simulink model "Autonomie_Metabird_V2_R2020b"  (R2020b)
settings: Solver=VariableStepAuto  StartTime=0.0  StopTime=450  RelTol=1e-3
model workspace (MAT data in the model file):
  Q = 1
undefined symbols (not defined in the file): set
libraries: fl_lib x7, nesl_utility x5, ee_lib x2

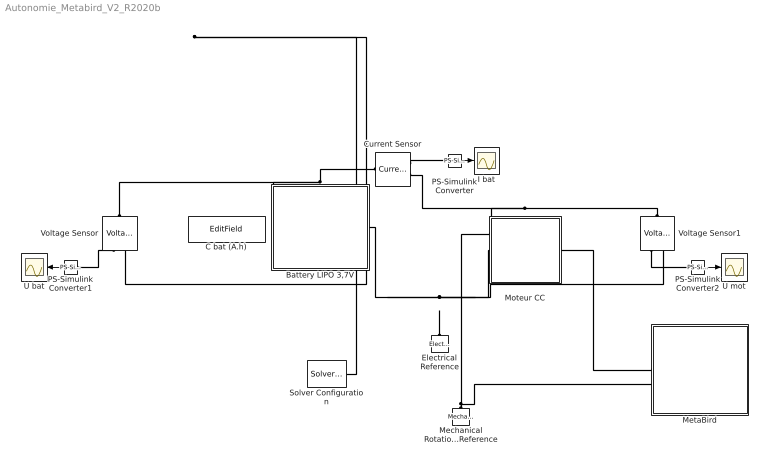
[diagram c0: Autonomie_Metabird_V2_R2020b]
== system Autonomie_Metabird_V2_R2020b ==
  Battery LIPO 3,7V : Subsystem
  C bat (A.h) : EditField  Description=EEE  LabelPosition=Hide  ShowInitialText=on  Alignment=Center
  Current Sensor : fl_lib/Electrical/Electrical Sensors/Current Sensor
  Electrical Reference : fl_lib/Electrical/Electrical Elements/Electrical Reference
  I bat : Scope
  Mechanical Rotational Reference : fl_lib/Mechanical/Rotational Elements/Mechanical Rotational Reference
  MetaBird : Subsystem
  Moteur CC : Subsystem
  PS-Simulink Converter : nesl_utility/PS-Simulink Converter  PhysicalDomain=network_engine_domain  SubClassName=ps_output  LeftPortType=input  RightPortType=output  PseudoPeriodic=off  Frequencies=[]  Unit=mA  AffineConversion=off
  PS-Simulink Converter1 : nesl_utility/PS-Simulink Converter  PhysicalDomain=network_engine_domain  SubClassName=ps_output  LeftPortType=input  RightPortType=output  PseudoPeriodic=off  Frequencies=[]  Unit=V  AffineConversion=off
  PS-Simulink Converter2 : nesl_utility/PS-Simulink Converter  PhysicalDomain=network_engine_domain  SubClassName=ps_output  LeftPortType=input  RightPortType=output  PseudoPeriodic=off  Frequencies=[]  Unit=V  AffineConversion=off
  Solver Configuration : nesl_utility/Solver Configuration  PhysicalDomain=network_engine_domain  SubClassName=solver  LeftPortType=input  RightPortType=generic  Tones=[]  Harmonics=[]  SimulateNoise=off  Profile=off  UseLocalSampling=off  EnableSwitchedLinearOptims=on  FrequencyDomain=off  UseCCode=off  RelTol=0.001  AbsTol=0.001  MinStep=1e-09  ToWorkspace=off  RevertToSquareIcSolve=off  NumHomotopyIterations=100  PhasorMode=off  PhasorModeNumHarmonics=1  DoDC=off  ResidualTolerance=1e-09  UseLocalSolver=off  LocalSolverChoice=NE_BACKWARD_EULER_ADVANCER  LocalSolverSampleTime=0.001  DoFixedCost=off  MaxNonlinIter=3  MaxModeIter=2  ComputeImpulses=off  ImpulseIterations=2  LinearAlgebra=auto  EquationFormulation=NE_TIME_EF  DelaysMemoryBudget=1024  AutomaticFiltering=on  FilteringTimeConstant=0.001  PartitionStorageMethod=AS_NEEDED  PartitionMemoryBudget=1024  PartitionMethod=ROBUST
  U bat : Scope
  U mot : Scope
  Voltage Sensor : fl_lib/Electrical/Electrical Sensors/Voltage Sensor
  Voltage Sensor1 : fl_lib/Electrical/Electrical Sensors/Voltage Sensor
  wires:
  PS-Simulink Converter/1 -> I bat/1
  PS-Simulink Converter1/1 -> U bat/1
  PS-Simulink Converter2/1 -> U mot/1
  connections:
  Voltage Sensor/LConn1 -- Current Sensor/LConn1 -- Battery LIPO 3,7V/LConn1
  Voltage Sensor1/LConn1 -- Moteur CC/LConn3 -- Current Sensor/RConn2
  Electrical Reference/LConn1 -- Voltage Sensor1/RConn2 -- Moteur CC/LConn2 -- Voltage Sensor/RConn2 -- Solver Configuration/RConn1 -- Battery LIPO 3,7V/RConn1
  Current Sensor/RConn1 -- PS-Simulink Converter/LConn1
  PS-Simulink Converter1/LConn1 -- Voltage Sensor/RConn1
  Voltage Sensor1/RConn1 -- PS-Simulink Converter2/LConn1
  Moteur CC/RConn1 -- MetaBird/LConn1
  Mechanical Rotational Reference/LConn1 -- MetaBird/LConn2 -- Moteur CC/LConn1

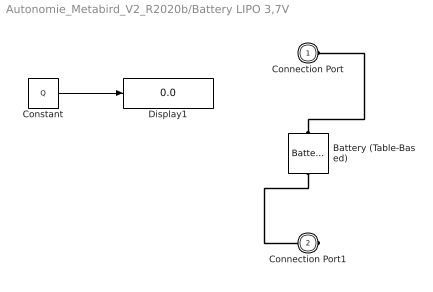
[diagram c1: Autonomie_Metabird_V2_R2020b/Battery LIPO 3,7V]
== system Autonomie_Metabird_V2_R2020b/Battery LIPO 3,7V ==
  Battery (Table-Based) : ee_lib/Sources/Battery (Table-Based)  Tag={'toolbox/physmod/elec/library/m/ee_lib_parts';'Sources/Battery__Table_Based_/Korea_Powercell/PD3032.xml'}  SOC_vec="[0 0.01 0.02 0.03 0.04 0.05 0.06 0.07 0.08 0.09 0.1 0.11 0.12 0.13 0.14 0.15 0.16 0.17 0.18 0.19 0.2 0.21 0.22 0.23 0.24 0.25 0.26 0.27 0.28 0.29 0.3 0.31 0.32 0.33 0.34 0.35 0.36 0.37 0.38 0.39 0.4 0.41 0.42 0.43 0.44 0.45 0.46 0.47 0.48 0.49 0.5 0.51 0.52 0.53 0.54 0.55 0.56 0.57 0.58 0.59 0.6 0.61 0.62 0.63 0.64 0.65 0.66 0.67 0.68 0.69 0.7 0.71 0.72 0.73 0.74 0.75 0.76 0.77 0.78 0.79 0.8 0.81 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"  T_dependence=ee.enum.temperature_dependence.no  prm_dir=ee.enum.battery.prm_dir.noCurrentDirectionality  T_vec=[-20 -10 25] degC  V0_mat=[2.95724 3.3564 3.49366 3.58258 3.63766 3.68332 3.70873 3.73055 3.74166 3.74045 3.73776 3.73631 3.73521 3.73661 3.73787 3.73862 3.74076 3.74303 3.74502 3.7472 3.74981 3.75229 3.7538 3.75584 3.75779 3.75969 3.76148 3.76318 3.76489 3.76695 3.76868 3.77025 3.77183 3.77343 3.77506 3.77658 3.77841 3.78029 3.78217 3.78415 3.78659 3.78921 3.79241 3.7956 3.79881 3.80207 3.80534 3.80863 3.81212 3.81572 3.8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  V0_vec=[2.95724 3.3564 3.49366 3.58258 3.63766 3.68332 3.70873 3.73055 3.74166 3.74045 3.73776 3.73631 3.73521 3.73661 3.73787 3.73862 3.74076 3.74303 3.74502 3.7472 3.74981 3.75229 3.7538 3.75584 3.75779 3.75969 3.76148 3.76318 3.76489 3.76695 3.76868 3.77025 3.77183 3.77343 3.77506 3.77658 3.77841 3.78029 3.78217 3.78415 3.78659 3.78921 3.79241 3.7956 3.79881 3.80207 3.80534 3.80863 3.81212 3.81572 3.8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  R0_mat=[0.86823 1.97565 2.19839 2.30336 2.32493 2.32311 2.27325 2.21593 2.13322 2.00795 1.88032 1.79212 1.70777 1.65332 1.59953 1.54628 1.51052 1.47625 1.44119 1.41044 1.38852 1.36656 1.34119 1.32173 1.30512 1.28839 1.27179 1.25526 1.23874 1.2262 1.21367 1.20059 1.1875 1.17438 1.1611 1.14754 1.13738 1.12789 1.11839 1.10879 1.10081 1.09337 1.08812 1.08292 1.0777 1.07242 1.06713 1.0619 1.0576 1.05404 1.051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  R0_vec=[0.86823 1.97565 2.19839 2.30336 2.32493 2.32311 2.27325 2.21593 2.13322 2.00795 1.88032 1.79212 1.70777 1.65332 1.59953 1.54628 1.51052 1.47625 1.44119 1.41044 1.38852 1.36656 1.34119 1.32173 1.30512 1.28839 1.27179 1.25526 1.23874 1.2262 1.21367 1.20059 1.1875 1.17438 1.1611 1.14754 1.13738 1.12789 1.11839 1.10879 1.10081 1.09337 1.08812 1.08292 1.0777 1.07242 1.06713 1.0619 1.0576 1.05404 1.051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  R0_dis_mat=[0.03 0.015 0.002;0.04 0.017 0.008;0.039 0.012 0.006;0.027 0.013 0.021] % Parameter not set Ohm  R0_dis_vec=[0.015 0.017 0.012 0.013] % Parameter not set Ohm  R0_ch_mat=[0.03 0.015 0.002;0.04 0.017 0.008;0.039 0.012 0.006;0.027 0.013 0.021] % Parameter not set Ohm  R0_ch_vec=[0.015 0.017 0.012 0.013] % Parameter not set Ohm  AH_vec=[0.058 0.058 0.058] hr*A  AH=Q+Q*0.15 hr*A  prm_leak=ee.enum.battery.prm_leak.disabled  Rleak_vec=[8000 7000 6000] % Parameter not set Ohm  Rleak=7000 % Parameter not set Ohm  extrapolation_option=ee.enum.extrapolation.nearest  prm_dyn=ee.enum.battery.prm_dyn.off  R1_mat=[0.089 0.076 0.01;0.042 0.022 0.099;0.019 0.007 0.002;0.051 0.043 0.029] % Parameter not set Ohm  R1_vec=[0.076 0.022 0.007 0.043] % Parameter not set Ohm  tau1_mat=[44 148 235;93 110 1000;19 27 133;0.5 22 3] % Parameter not set s  tau1_vec=[148 110 27 22] % Parameter not set s  R2_mat=[0.014 0.382 0.407;0.028 0.006 0.007;0.014 0.007 0.006;0.333 0.956 0.912] % Parameter not set Ohm  R2_vec=[0.382 0.006 0.007 0.956] % Parameter not set Ohm  tau2_mat=[1 44 5644;11 24 506;2 14 330;3310 13419 30216] % Parameter not set s  tau2_vec=[44 24 14 13419] % Parameter not set s  R3_mat=[0.014 0.382 0.407;0.028 0.006 0.007;0.014 0.007 0.006;0.333 0.956 0.912] % Parameter not set Ohm  R3_vec=[0.382 0.006 0.007 0.956] % Parameter not set Ohm  tau3_mat=[1 44 5644;11 24 506;2 14 330;3310 13419 30216] % Parameter not set s  tau3_vec=[44 24 14 13419] % Parameter not set s  R4_mat=[0.014 0.382 0.407;0.028 0.006 0.007;0.014 0.007 0.006;0.333 0.956 0.912] % Parameter not set Ohm  R4_vec=[0.382 0.006 0.007 0.956] % Parameter not set Ohm  tau4_mat=[1 44 5644;11 24 506;2 14 330;3310 13419 30216] % Parameter not set s  tau4_vec=[44 24 14 13419] % Parameter not set s  R5_mat=[0.014 0.382 0.407;0.028 0.006 0.007;0.014 0.007 0.006;0.333 0.956 0.912] % Parameter not set Ohm  R5_vec=[0.382 0.006 0.007 0.956] % Parameter not set Ohm  tau5_mat=[1 44 5644;11 24 506;2 14 330;3310 13419 30216] % Parameter not set s  tau5_vec=[44 24 14 13419] % Parameter not set s  prm_fade=ee.enum.battery.prm_fade.tableN  N0=100 % Parameter not set  dV0=0 % Parameter not set  dR0=0 % Parameter not set  dAH=0 % Parameter not set  dRleak=0 % Parameter not set  dR1=0 % Parameter not set  dR2=0 % Parameter not set  dR3=0 % Parameter not set  dR4=0 % Parameter not set  dR5=0 % Parameter not set  N0vec=[1 7 13 19 25 31 37 43 49 55 61 67 73 79 85 91 97 103 109 115 121 127 133 139 145 151 157 163 169 175 181 187 193 199 205 211 217 223 229 235 241 247 253 259 265 271 277 283 289 295 301 307 313 319 325 331 337 343 349 355 361 367 373 379 385 391 397 403 409 415 421 427 433 439 445 451 457 463 469 475 481 487 493 499]  Tfadevec=[298.15 323.15] % Parameter not set K  dV0vec=[0 -0.0628438826149197 -0.125687765229839 -0.18853164784478 -0.251375530459721 -0.314219413074662 -0.377063295689582 -0.451508979909996 -0.562003276816908 -0.667452593509906 -0.772901910202884 -0.878351226895861 -0.96290491111089 -1.04466751936566 -1.12332313736417 -1.20197875536267 -1.26256181580412 -1.3222060579416 -1.38185030007906 -1.44149454221653 -1.50255421857852 -1.56371974345091 -1.624885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  dR0vec=[0;0;0;0;0;0;0;0;0;0;0;0;0;0;0;0;0;0;0;0;0;0;0;0;0;0;0;0;0;0;0;0;0;0;0;0;0;0;0;0;0;0;0;0;0;0;0;0;0;0;0;0;0;0;0;0;0;0;0;0;0;0;0;0;0;0;0;0;0;0;0;0;0;0;0;0;0;0;0;0;0;0;0;0] % Parameter not set  dAHvec=[0 -0.130046736538462 -0.260093473076939 -0.39014020961543 -0.520186946153922 -0.650233682692399 -0.780280419230876 -0.934335482021324 -1.19380012181077 -1.45326476160023 -1.71272940138966 -1.9721940411791 -2.23165868096855 -2.49022842430935 -2.73897248216537 -2.9877165400214 -3.23646059787742 -3.48520465573346 -3.73394871358948 -3.9826927714455 -4.23143682930151 -4.48018088715753 -4.7289249450135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  dRleakvec=[0 0 0] % Parameter not set  dR1vec=[0 0 0] % Parameter not set  dR2vec=[0 0 0] % Parameter not set  dR3vec=[0 0 0] % Parameter not set  dR4vec=[0 0 0] % Parameter not set  dR5vec=[0 0 0] % Parameter not set  dV0mat=[0 0;0 0;0 0] % Parameter not set  dR0mat=[0 0;0 0;0 0] % Parameter not set  dAHmat=[0 0;0 0;0 0] % Parameter not set  dRleakmat=[0 0;0 0;0 0] % Parameter not set  dR1mat=[0 0;0 0;0 0] % Parameter not set  dR2mat=[0 0;0 0;0 0] % Parameter not set  dR3mat=[0 0;0 0;0 0] % Parameter not set  dR4mat=[0 0;0 0;0 0] % Parameter not set  dR5mat=[0 0;0 0;0 0] % Parameter not set  temperature=298.15 K  i_specify=off  i_priority=None  i=0 A  i_nominal_specify=off  i_nominal_unit=A  i_nominal_value=1  v_specify=off  v_priority=None  v=0 V  v_nominal_specify=off  v_nominal_unit=V  v_nominal_value=1  stateOfCharge_specify=on  stateOfCharge_priority=High  stateOfCharge=1  stateOfCharge_nominal_specify=off  stateOfCharge_nominal_unit=1  stateOfCharge_nominal_value=1  num_cycles_specify=off  num_cycles_priority=High  num_cycles=0  num_cycles_nominal_specify=off  num_cycles_nominal_unit=1  num_cycles_nominal_value=1  thermal_mass=30000 J/K  temperature_specify=off  temperature_priority=High  temperature_nominal_specify=off  temperature_nominal_unit=K  temperature_nominal_value=1
  Constant : Constant  Value=Q
  Display1 : Display
  Connection Port : PMIOPort  Side=Left
  Connection Port1 : PMIOPort  Port=2  Side=Right
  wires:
  Constant/1 -> Display1/1
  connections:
  Battery (Table-Based)/RConn1 -- Connection Port1/RConn1
  Battery (Table-Based)/LConn1 -- Connection Port/RConn1

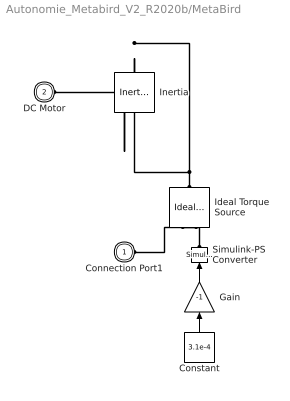
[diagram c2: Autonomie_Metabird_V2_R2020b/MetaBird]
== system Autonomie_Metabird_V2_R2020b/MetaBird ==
  Constant : Constant  Value=3.1e-4
  Gain : Gain  Gain=-1
  Ideal Torque Source : fl_lib/Mechanical/Mechanical Sources/Ideal Torque Source
  Inertia : fl_lib/Mechanical/Rotational Elements/Inertia  inertia=1.91e-8 kg*m^2  num_ports=foundation.enum.numPorts2.one  w_specify=off  w_priority=High  w=0 rad/s  w_nominal_specify=off  w_nominal_unit=rad/s  w_nominal_value=1  t_specify=off  t_priority=None  t=0 N*m  t_nominal_specify=off  t_nominal_unit=N*m  t_nominal_value=1
  Simulink-PS Converter : nesl_utility/Simulink-PS Converter  PhysicalDomain=network_engine_domain  SubClassName=ps_input  LeftPortType=input  RightPortType=output  PseudoPeriodic=off  Frequencies=[]  NoiseDistribution=none  NoiseParameters=[]  Unit=N*m  AffineConversion=off  FilteringAndDerivatives=provide  SimscapeFilterOrder=1  InputFilterTimeConstant=0.001  UdotUserProvided=0
  Connection Port1 : PMIOPort  Side=Left
  DC Motor : PMIOPort  Port=2  Side=Left
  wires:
  Constant/1 -> Gain/1
  Gain/1 -> Simulink-PS Converter/1
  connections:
  Ideal Torque Source/LConn1 -- DC Motor/RConn1 -- Inertia/LConn1
  Simulink-PS Converter/RConn1 -- Ideal Torque Source/RConn1
  Connection Port1/RConn1 -- Ideal Torque Source/RConn2

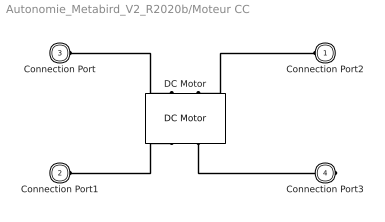
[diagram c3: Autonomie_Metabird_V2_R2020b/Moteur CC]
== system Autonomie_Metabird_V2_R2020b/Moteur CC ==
  DC Motor : ee_lib/Electromechanical/Brushed Motors/DC Motor  field_option=ee.enum.field_option.pm  Rf=100 Ohm  Lf=1 H  Laf=0.15 H  If0=0 A  parameterization=ee.enum.dcparam_option.load_speed  Ra=3.9 Ohm  La=12e-6 H  emf_or_torque=ee.enum.emf_or_torque.kv  Kv=0.072e-3 V/rpm  Ki=6.876e-4 N*m/A  T_stall=0.24e-3 N*m  w_max=53000 rpm  w_rated=37000 rpm  P_rated=1.6 W  V_rated=3.7 V  J=0 g*cm^2  lam_param=ee.enum.lam_param.current  lam=0 N*m/(rad/s)  i_noload=68.1 mA  V_i_noload=3.7 V  speed0=0 rpm  enable_fault_armature=ee.enum.faults.faultEnable.no  rev_faulted=1 / 3  G_faulted_armature=1e-5 S  fault_trigger_armature=ee.enum.faults.faultTrigger.temporal  t_fault_armature=1 s  max_permissible_current_armature=inf A  t_fail_on_current_armature=1 s  enable_fault_field=ee.enum.faults.faultEnable.no  G_faulted_field=1e-5 S  fault_trigger_field=ee.enum.faults.faultTrigger.temporal  t_fault_field=1 s  max_permissible_current_field=inf A  t_fail_on_current_field=1 s  fault_action=ee.enum.faults.faultAction.none  alpha=3.93e-3 1/K  Tmeas=25 degC  thermal_mass=100 J/K  initial_temperature=25 degC
  Connection Port2 : PMIOPort  Side=Left
  Connection Port1 : PMIOPort  Port=2  Side=Left
  Connection Port : PMIOPort  Port=3  Side=Left
  Connection Port3 : PMIOPort  Port=4  Side=Right
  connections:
  Connection Port/RConn1 -- DC Motor/LConn1
  Connection Port1/RConn1 -- DC Motor/RConn1
  Connection Port2/RConn1 -- DC Motor/LConn2
  DC Motor/RConn2 -- Connection Port3/RConn1
